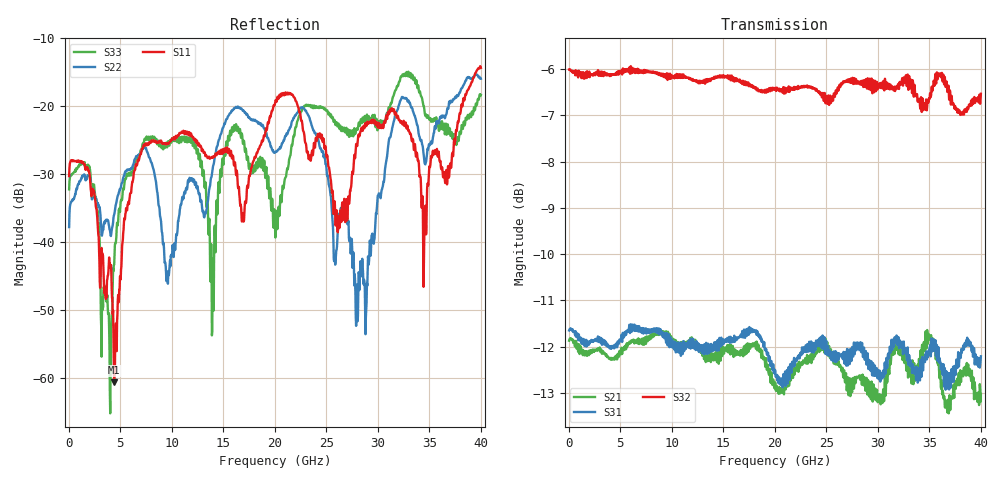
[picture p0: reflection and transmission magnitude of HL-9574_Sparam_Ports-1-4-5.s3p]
# GHZ S RI R 50.0
!; PortSelection: Port_123
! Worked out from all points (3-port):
!   1143 points, 35 MHz to 40.01 GHz, reference 50 ohm
!   strongest paths, dB at 35 MHz, 10.01 GHz, 20.02 GHz, 30.03 GHz, 40.01 GHz:
!     S32: -6.0, -6.1, -6.4, -6.3, -6.5
!     S31: -11.7, -11.8, -12.5, -12.5, -12.2
!     S21: -11.9, -12.0, -12.8, -13.1, -13.0
!   lowest |S11| = -60.7 dB at 4.41 GHz (marker M1), VSWR 1.00, Z = 50.1 + j0.0225 ohm
!   |S11| at or under -10 dB: start of sweep to end of sweep
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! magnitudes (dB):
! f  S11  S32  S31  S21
! 35 MHz  -30.3  -6.0  -11.7  -11.9
! 4.41 GHz  -60.7  -6.1  -12.0  -12.3
! 7.28 GHz  -25.7  -6.1  -11.7  -11.9
! 9.59 GHz  -25.5  -6.2  -12.0  -11.7
! 13.89 GHz  -27.5  -6.2  -12.1  -12.2
! 20.02 GHz  -19.6  -6.4  -12.5  -12.8
! 28.8 GHz  -22.5  -6.4  -12.1  -13.0
! 32.2 GHz  -22.4  -6.3  -11.9  -12.1
! 34.55 GHz  -38.0  -6.7  -12.3  -12.1
! 40.01 GHz  -14.3  -6.5  -12.2  -13.0
